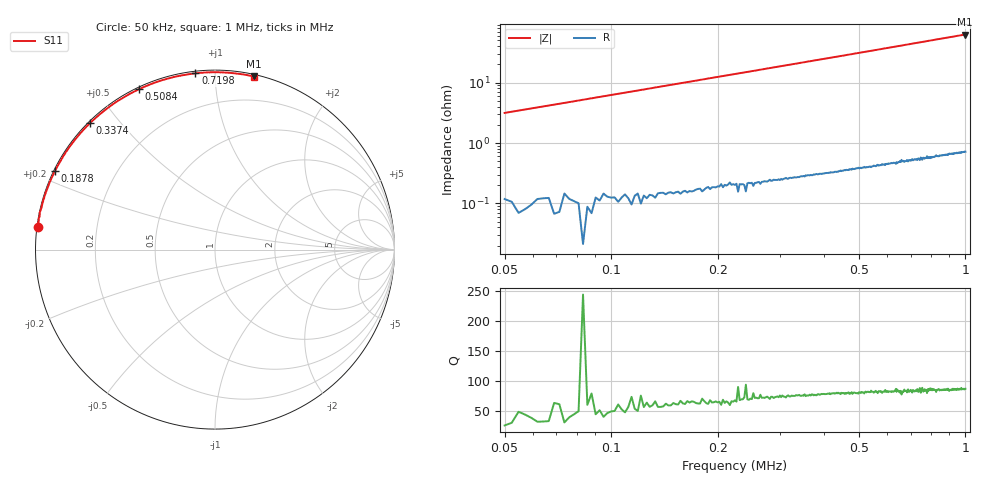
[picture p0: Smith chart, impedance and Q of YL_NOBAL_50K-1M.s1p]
!File
# Hz S RI R 50
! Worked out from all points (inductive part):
!   401 points, 50 kHz to 1 MHz, reference 50 ohm
!   read as one part to ground: L = 9.95 uH near 54.75 kHz
!   highest Q = 87.4 at 997.6 kHz (marker M1), where L = 9.97 uH
!   S11 on the Smith chart (normalised r, x): 50 kHz: 0.00, +0.06; 187.8 kHz: 0.00, +0.23; 337.4 kHz: 0.01, +0.42; 508.4 kHz: 0.01, +0.63; 719.8 kHz: 0.01, +0.89; 1 MHz: 0.01, +1.25
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50000  -0.9874 0.1248
54750  -0.9878 0.1366
88000  -0.9735 0.2166
126000  -0.9473 0.3051
168750  -0.9101 0.3996
187750  -0.8903 0.4395
237625  -0.8335 0.539
263750  -0.8003 0.5868
287500  -0.7673 0.6275
311250  -0.7336 0.666
337375  -0.6954 0.7057
373000  -0.641 0.7546
406250  -0.589 0.7955
453750  -0.5134 0.8457
482250  -0.4677 0.8715
508375  -0.426 0.8926
525000  -0.3995 0.9045
558250  -0.3471 0.926
589125  -0.2996 0.9421
643750  -0.2174 0.9644
677000  -0.1695 0.9737
719750  -0.1095 0.982
762500  -0.0517 0.9867
821875  0.0241 0.988
881250  0.0938 0.984
938250  0.1565 0.9761
997625  0.2169 0.9648
1000000  0.2192 0.9643
